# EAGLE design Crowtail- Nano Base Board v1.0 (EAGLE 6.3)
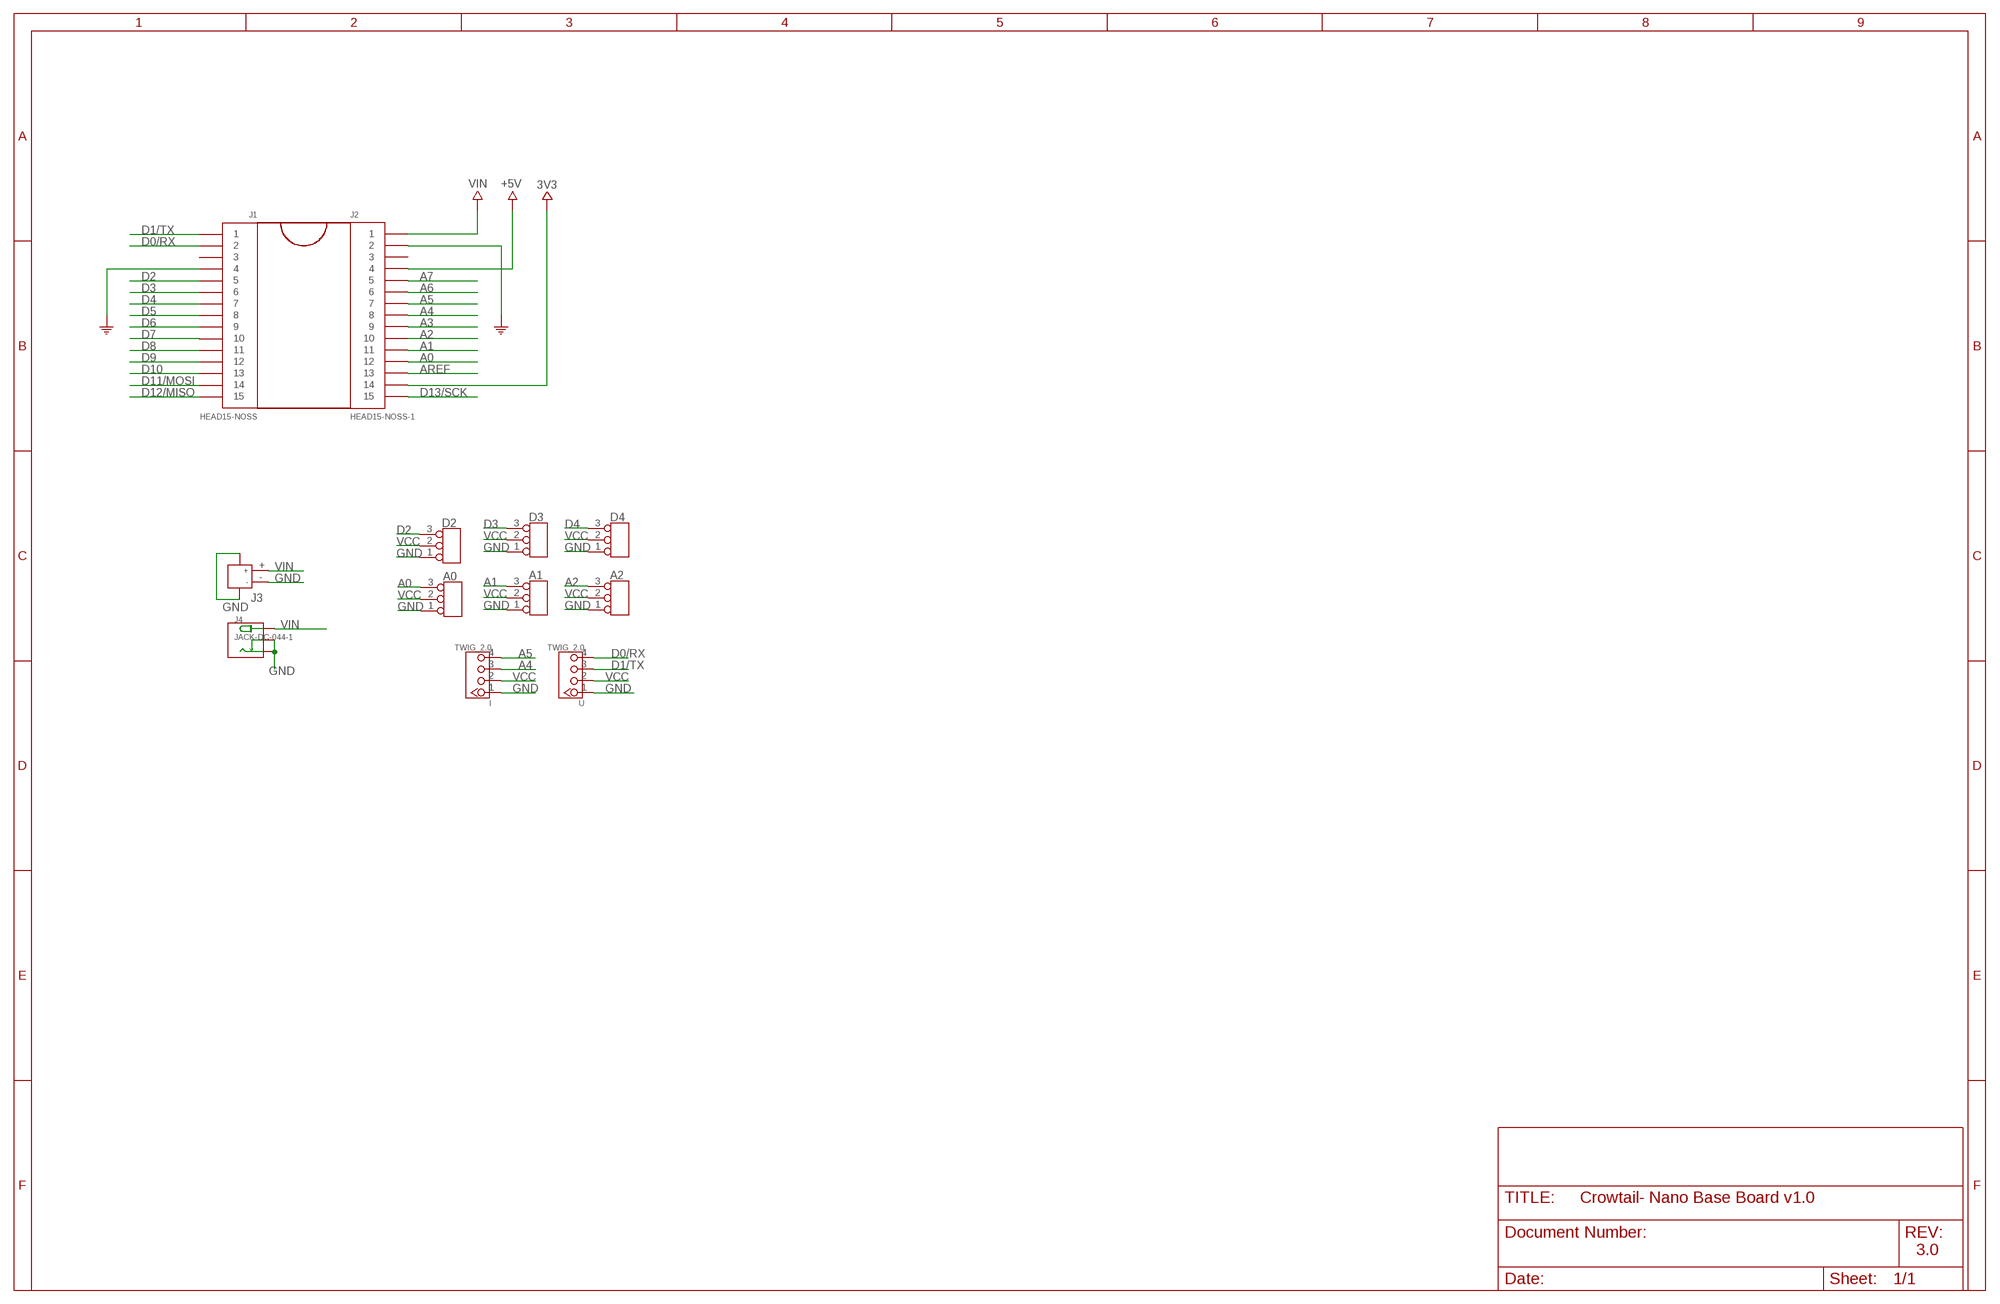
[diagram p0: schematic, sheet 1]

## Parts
A0  TINKER_3P_DIP  [3P_2.0_DIP]
A1  TINKER_3P_DIP  [3P_2.0_DIP]
A2  TINKER_3P_DIP  [3P_2.0_DIP]
D2  TINKER_3P_DIP  [3P_2.0_DIP]
D3  TINKER_3P_DIP  [3P_2.0_DIP]
D4  TINKER_3P_DIP  [3P_2.0_DIP]
I  TWIG_2.0  [2.0_1X4]
J1  HEAD15-NOSS  [HEAD15-NOSS]
J2  HEAD15-NOSS-1  [HEAD15-NOSS-1]
J3  JACK-JST-2P-SMD-PW'2.0'  [JST-SMD-2.0-90D]
J4  JACK-DC-044-1  [DC-404-1]
U  TWIG_2.0  [2.0_1X4]

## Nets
3V3: J2.14
A0: A0.3 J2.12
A1: A1.3 J2.11
A2: A2.3 J2.10
A3: J2.9
A4: I.3 J2.8
A5: I.4 J2.7
A6: J2.6
A7: J2.5
AREF: J2.13
D0/RX: J1.2 U.4
D1/TX: J1.1 U.3
D2: D2.3 J1.5
D3: D3.3 J1.6
D4: D4.3 J1.7
D5: J1.8
D6: J1.9
D7: J1.10
D8: J1.11
D9: J1.12
D10: J1.13
D11/MOSI: J1.14
D12/MISO: J1.15
D13/SCK: J2.15
GND: A0.1 A1.1 A2.1 D2.1 D3.1 D4.1 I.1 J1.4 J2.2 J3.3 J3.4 J3.- J4.- J4.CDN U.1 ; supply symbol labelled COM
VCC: A0.2 A1.2 A2.2 D2.2 D3.2 D4.2 I.2 J2.4 U.2 ; supply symbol labelled +5V
VIN: J2.1 J3.+ J4.+
Unconnected: J1.3 J2.3

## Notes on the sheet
- 3.0

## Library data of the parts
A0 A1 A2 D2-D4 = Connector:TINKER_3P_DIP
I U = CONNECTER:TWIG_2.0
J1 = MyCON2:HEAD15-NOSS
J2 = MyCON2:HEAD15-NOSS-1
J3 = Connector:JACK-JST-2P-SMD-PW
J4 = Connector:JACK-DC-044-1

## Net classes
0 default: width 0.003 mm, drill 0.254 mm, clearance 0.152 mm
2 gnd: width 0.305 mm, drill 0.559 mm, clearance 0.254 mm

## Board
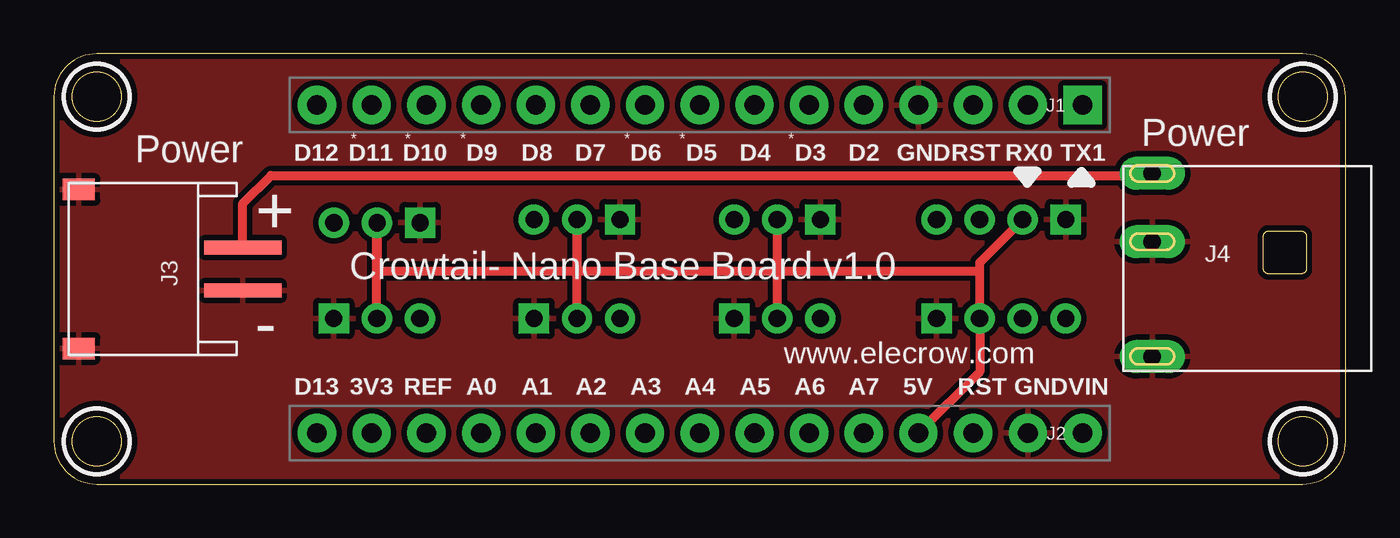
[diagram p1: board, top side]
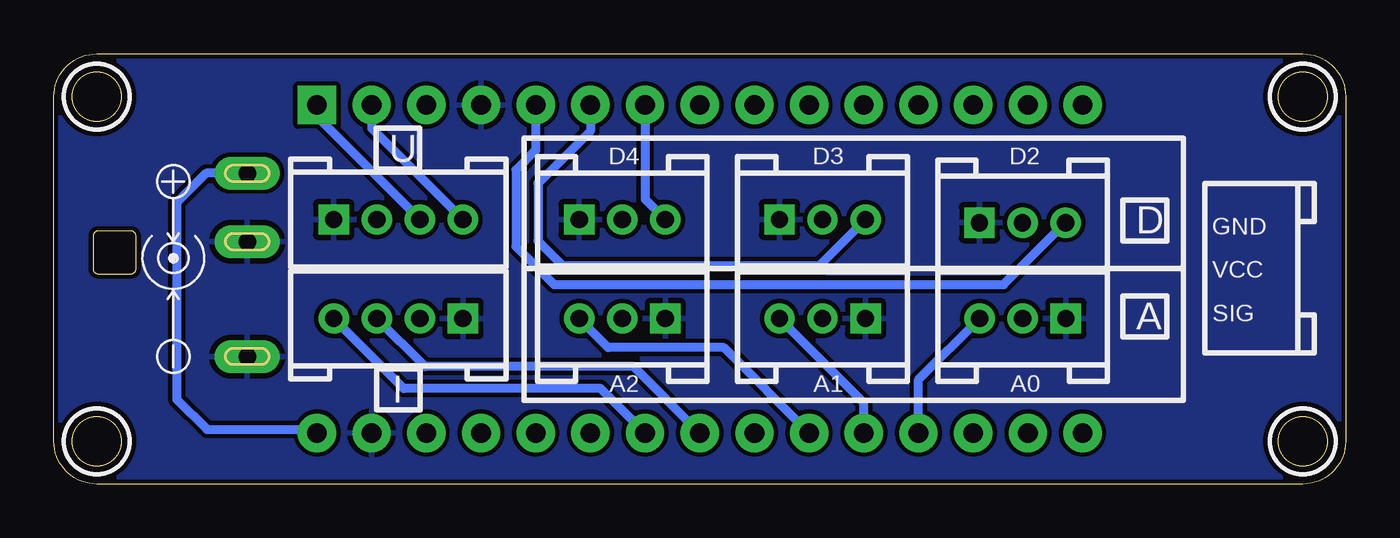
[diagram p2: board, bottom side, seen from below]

Size 60 x 20 mm. Coordinates in mm from the lower left corner, seen from the top.
Outline: 58,20 2,20 arc90 0,18 0,2 arc90 2,0 58,0 arc90 60,2 60,18 arc90 58,20
Outline: circle at 58,18 radius 1.14
Outline: circle at 58,2 radius 1.14
Outline: circle at 2,18 radius 1.14
Outline: circle at 2,2 radius 1.14
Copper layers (1*16): Top 0.035mm / dielectric 1.5mm / Bottom 0.035mm
Design rules "default *": minimum track width 8mil, minimum drill 16mil, track to track 8mil, track to pad 8mil, pad to pad 8mil, via to via 8mil, smd to smd 8mil, copper to edge 8mil, drill to drill 8mil, minimum pad ring 12mil, minimum via ring 8mil, stop-mask expansion 4mil, vias tented up to drill 18mil, thermal gap 10mil
tRestrict: area 56.5,16.5 to 59.5,19.5; area 56.5,0.5 to 59.5,3.5; area 0.5,16.5 to 3.5,19.5; area 0.5,0.5 to 3.5,3.5
bRestrict: area 56.5,16.5 to 59.5,19.5; area 56.5,0.5 to 59.5,3.5; area 0.5,16.5 to 3.5,19.5; area 0.5,0.5 to 3.5,3.5

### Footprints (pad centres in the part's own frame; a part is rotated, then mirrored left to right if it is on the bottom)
3P_2.0_DIP = drill 0.8 pad 1.27 square: 1 -2,0 | drill 0.8 pad 1.27: 2 0,0; 3 2,0
2.0_1X4 = drill 0.8 pad 1.27 square: 1 -3,0 | drill 0.8 pad 1.27: 2 -1,0; 3 1,0; 4 3,0
HEAD15-NOSS = drill 0.914 pad 1.778 square: 1 0,0 | drill 0.914 pad 1.778: 2 2.54,0; 3 5.08,0; 4 7.62,0; 5 10.16,0; 6 12.7,0; 7 15.24,0; 8 17.78,0; 9 20.32,0; 10 22.86,0; 11 25.4,0; 12 27.94,0; 13 30.48,0; 14 33.02,0; 15 35.56,0
HEAD15-NOSS-1 = drill 0.914 pad 1.778: 1 0,0; 2 2.54,0; 3 5.08,0; 4 7.62,0; 5 10.16,0; 6 12.7,0; 7 15.24,0; 8 17.78,0; 9 20.32,0; 10 22.86,0; 11 25.4,0; 12 27.94,0; 13 30.48,0; 14 33.02,0; 15 35.56,0
JST-SMD-2.0-90D = smd 1 x 1.5: 3 3.7,-2.54; 4 -3.7,-2.54 | smd 0.635 x 3.6: + -1,5.08; - 1,5.08
DC-404-1 = drill 0.813 pad 1.524 long: + 4.445,5.08; - -4.064,5.08; CDN 1.27,5.08

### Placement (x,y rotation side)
A0  15,7.7 180 bottom
A1  24.3,7.7 180 bottom
A2  33.6,7.7 180 bottom
D2  15.01,12.15 0 bottom
D3  24.3,12.3 0 bottom
D4  33.6,12.3 0 bottom
I  44,7.7 180 bottom
J1  47.78,17.62 180 top
J2  47.78,2.38 180 top
J3  3.7,10 270 top
J4  56.1,10 90 top
U  44,12.3 0 bottom

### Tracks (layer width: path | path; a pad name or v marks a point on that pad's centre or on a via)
A0
  Bottom 0.406: J2.12 19.84,4.86 A0.3
A1
  Bottom 0.406: J2.11 22.38,3.78 A1.3
A2
  Bottom 0.406: J2.10 28.89,6.35 34.25,6.35 A2.3
A4
  Bottom 0.406: J2.8 33.08,5.46 42.76,5.46 I.3
A5
  Bottom 0.406: J2.7 34.6,4.45 43.74,4.45 I.4
D0/RX
  Bottom 0.406: J1.2 45.24,16.54 U.4
D1/TX
  Bottom 0.406: J1.1 47.78,17.08 U.3
D2
  Bottom 0.406: J1.5 37.62,15.52 38.54,14.61 38.54,11.05 36.76,9.27 15.89,9.27 D2.3
D3
  Bottom 0.406: J1.6 35.08,16.41 37.52,13.97 37.52,11.3 36.38,10.16 24.44,10.16 D3.3
D4
  Bottom 0.406: J1.7 32.54,13.24 D4.3
GND
  pour Top (isolate 0.254): -0.27,20.13 60.25,20.15 60.06,-0.11 -0.46,-0.13
  pour Bottom (isolate 0.203): -0.33,20.11 60.1,20.07 60.04,-0.09 -0.39,-0.05
VCC
  Top 0.406: A0.2 D2.2 15.01,9.94 15.04,9.91 24.3,9.91 | A1.2 24.3,9.91 | 24.3,9.91 D3.2 24.3,9.92 24.31,9.91 33.47,9.91 33.6,10.03 | 33.6,10.03 A2.2 33.6,9.89 33.58,9.91 42.87,9.91 43,10.03 | 33.6,10.03 D4.2 | 43,10.03 I.2 43,5.22 J2.4 | 43,10.03 43,10.3 U.2
VIN
  Top 0.406: J3.+ 8.78,13.04 10.09,14.35 50.93,14.35 J4.+
  Bottom 0.406: J4.+ 52.92,14.45 54.28,13.08 54.28,3.94 52.89,2.54 47.94,2.54 J2.1

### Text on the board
tPlace: * | * | * | * | * | * | Power | Power | D12 | D11 | D10 | D9 | D8 | D7 | D6 | D5 | D4 | D3 | D2 | GND | RST | RX0 | TX1 | + | Crowtail- Nano Base Board v1.0 | - | www.elecrow.com | D13 | 3V3 | REF | A0 | A1 | A2 | A3 | A4 | A5 | A6 | A7 | 5V | RST | GND | VIN
bPlace: GND | VCC | SIG
bNames: U | D | A | I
